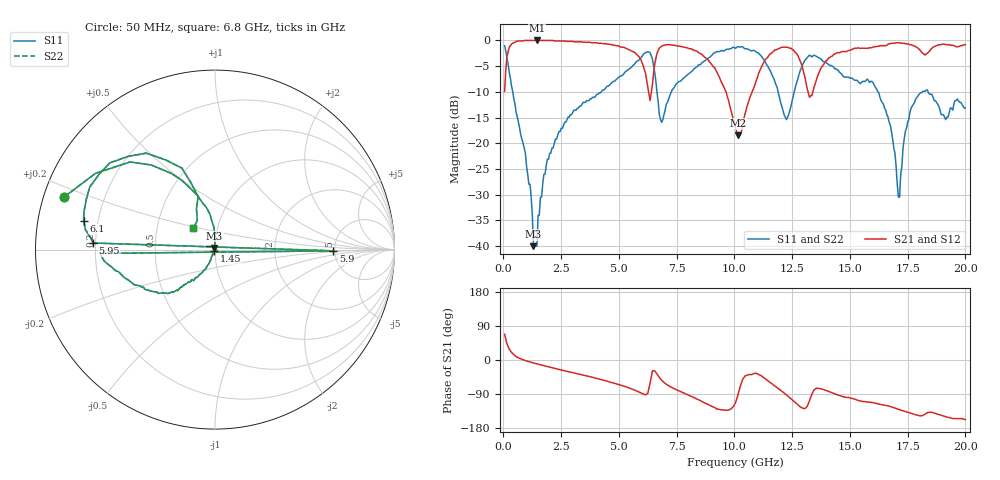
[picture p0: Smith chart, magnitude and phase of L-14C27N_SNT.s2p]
#	mhz	s	ma	r	50
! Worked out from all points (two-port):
!   400 points, 50 MHz to 20 GHz, reference 50 ohm
!   highest |S21| = 0.00 dB at 1.45 GHz (marker M1); lowest = -18.4 dB at 10.15 GHz (marker M2)
!   |S21| within 3 dB of the highest: 155.2 MHz to 5.83 GHz (5.675 GHz wide, 190 % of centre); 14.24 GHz to end of sweep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
!   lowest |S11| = -40.0 dB at 1.3 GHz (marker M3), VSWR 1.02, Z = 49.7 + j0.95 ohm
!   |S11| at or under -10 dB: 403.5 MHz to 4.231 GHz (3.828 GHz wide, 165 % of centre); 16.22 GHz to 18.13 GHz (1.913 GHz wide, 11.1 % of centre); 18.38 GHz to end of sweep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
!   |S22| runs from -40.0 to -1.0 dB; largest |S21 - S12| = 0
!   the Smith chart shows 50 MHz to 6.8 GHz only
!   S11 on the Smith chart (normalised r, x): 50 MHz: 0.06, +0.17; 1.45 GHz: 0.99, -0.01; 5.9 GHz: 4.88, -0.12; 5.95 GHz: 0.19, +0.03; 6.1 GHz: 0.14, +0.11; 6.8 GHz: 0.76, +0.19
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50  0.89 160.8  0.32 67.9  0.32 67.9  0.89 160.8
350  0.36 111.4  0.92 19.9  0.92 19.9  0.36 111.4
1300  0.01 107.2  1 -7.9  1 -7.9  0.01 107.2
1450  0.01 -134.5  1 -10.3  1 -10.3  0.01 -134.5
1900  0.07 -113.2  1 -17.2  1 -17.2  0.07 -113.2
3400  0.24 -129.6  0.97 -39.1  0.97 -39.1  0.24 -129.6
5850  0.64 -178.1  0.7 -84.1  0.7 -84.1  0.64 -178.1
5900  0.66 -0.6  0.68 -85.6  0.68 -85.6  0.66 -0.6
5950  0.68 176.9  0.65 -87.1  0.65 -87.1  0.68 176.9
6100  0.75 167.6  0.52 -90.9  0.52 -90.9  0.75 167.6
6700  0.25 114.4  0.8 -41.9  0.8 -41.9  0.25 114.4
6800  0.17 135.1  0.86 -49.8  0.86 -49.8  0.17 135.1
7300  0.33 -0.6  0.9 -73.0  0.9 -73.0  0.33 -0.6
7450  0.37 178.6  0.89 -77.4  0.89 -77.4  0.37 178.6
10050  0.84 110.3  0.14 -112.3  0.14 -112.3  0.84 110.3
10150  0.87 108.7  0.12 -93.3  0.12 -93.3  0.87 108.7
12250  0.17 83.9  0.86 -92.0  0.86 -92.0  0.17 83.9
13350  0.69 76.1  0.29 -90.4  0.29 -90.4  0.69 76.1
16700  0.16 -32.8  0.93 -121.8  0.93 -121.8  0.16 -32.8
17150  0.03 33.4  0.95 -131.4  0.95 -131.4  0.03 33.4
17950  0.29 72.3  0.84 -146.2  0.84 -146.2  0.29 72.3
20000  0.22 -86.8  0.91 -157.0  0.91 -157.0  0.22 -86.8
